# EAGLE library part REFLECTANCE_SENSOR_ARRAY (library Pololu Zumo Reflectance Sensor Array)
Zumo Reflectance Sensor Array Item #1419
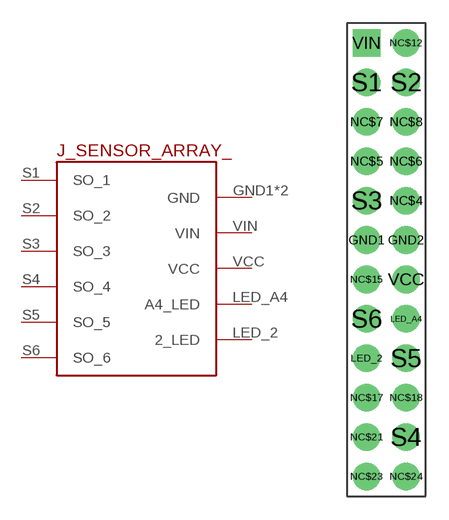
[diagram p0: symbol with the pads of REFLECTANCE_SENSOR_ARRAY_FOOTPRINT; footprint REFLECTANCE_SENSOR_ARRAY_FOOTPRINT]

Designator prefix J_SENSOR_ARRAY_

## REFLECTANCE_SENSOR_ARRAY  [REFLECTANCE_SENSOR_ARRAY_FOOTPRINT]
GND1  GND
GND2  GND
LED_2  2_LED
LED_A4  A4_LED
S1  SO_1
S2  SO_2
S3  SO_3
S4  SO_4
S5  SO_5
S6  SO_6
VCC  VCC
VIN  VIN

## Footprint REFLECTANCE_SENSOR_ARRAY_FOOTPRINT (pad centres in mm)
Zumo Reflectance Sensor Array Item #1419 Footprint
drill 0.9 pad 1.778: GND1 -1.27,0; GND2 1.27,0; LED_2 -1.27,-7.62; LED_A4 1.27,-5.08; NC$4 1.27,2.54; NC$5 -1.27,5.08; NC$6 1.27,5.08; NC$7 -1.27,7.62; NC$8 1.27,7.62; NC$12 1.27,12.7; NC$15 -1.27,-2.54; NC$17 -1.27,-10.16; NC$18 1.27,-10.16; NC$21 -1.27,-12.7; NC$23 -1.27,-15.24; NC$24 1.27,-15.24; S1 -1.27,10.16; S2 1.27,10.16; S3 -1.27,2.54; S4 1.27,-12.7; S5 1.27,-7.62; S6 -1.27,-5.08; VCC 1.27,-2.54
drill 0.9 pad 1.778 square: VIN -1.27,12.7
